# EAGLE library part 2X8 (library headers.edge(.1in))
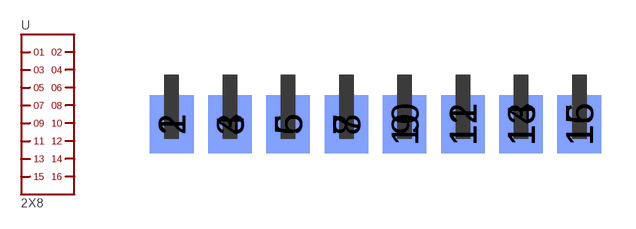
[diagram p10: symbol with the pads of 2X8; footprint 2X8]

Designator prefix -

## 2X8  [2X8]
1  1
2  2
3  3
4  4
5  5
6  6
7  7
8  8
9  9
10  10
11  11
12  12
13  13
14  14
15  15
16  16

## Footprint 2X8 (pad centres in mm)
smd 1.905 x 2.54: 1 0,-2.159; 3 2.54,-2.159; 5 5.08,-2.159; 7 7.62,-2.159; 9 10.16,-2.159; 11 12.7,-2.159; 13 15.24,-2.159; 15 17.78,-2.159
smd 1.905 x 2.54 bottom: 2 0,-2.159; 4 2.54,-2.159; 6 5.08,-2.159; 8 7.62,-2.159; 10 10.16,-2.159; 12 12.7,-2.159; 14 15.24,-2.159; 16 17.78,-2.159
